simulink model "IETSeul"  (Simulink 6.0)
settings: Solver=ode45  StartTime=0.0  StopTime=SimTime  FixedStep=1E-2  RelTol=1e-5
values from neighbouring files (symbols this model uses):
  beta = 1    [ResCourV1.m]    (also in ResCrV1.m; ResEnerV1.m; Constantes.m = 0.95; ConstantesBck.m = 0.95)
  Cdl = 731.3E-9    (= 7.313e-07)    [ResCourV1.m]    (also in ResCrV1.m; ResEnerV1.m; Constantes.m = 6.03e-07; ConstantesBck.m = 6.03e-07)
  Cmem = 1E-6*Sm*(1-b)    (= 2.826e-08)    [Constantes.m]    (also in ConstantesBck.m = 3.14e-11; ImpedanceZtissus.m = 4e-08; Ztissus.m = 4e-08; CalculCharge.m = 1)
  I0Stim = AddI    (= 0)    [WaveComp.m]    (also in WaveCompIET.m; WaveCompIETAnim.m; WaveCompIETIf.m; WaveCompIETSeul.m = Hm(i)*1E-6)
  Rcan = 6.398E3*Sm*(1-b)    (= 180.80748)    [Constantes.m]    (also in ConstantesBck.m = 0.03454; ImpedanceZtissus.m = 44; Ztissus.m = 44)
  Rct = 605.2E3    (= 605200)    [ResCourV1.m]    (also in ResCrV1.m; ResEnerV1.m; Constantes.m = 185600; ConstantesBck.m = 185600)
  sigma = 68000    [ResCourV1.m]    (also in ResCrV1.m; ResEnerV1.m; Constantes.m = 66466; ConstantesBck.m = 66466)
  T0Stim = i    [WaveComp.m]    (also in WaveCompIET.m; WaveCompIETAnim.m = 5; WaveCompIETIf.m; WaveCompIETSeul.m = T0Hm(i)*1E-3)
  TypeStim = 5    [WaveComp.m]    (also in WaveCompIET.m; WaveCompIETAnim.m; WaveCompIETIf.m; WaveCompIETSeul.m)
libraries: simulink x1

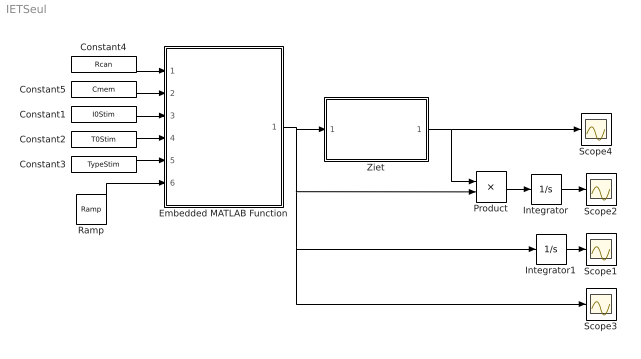
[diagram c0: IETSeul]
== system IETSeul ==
  Constant1 : Constant  Value=I0Stim
  Constant2 : Constant  Value=T0Stim
  Constant3 : Constant  Value=TypeStim
  Constant4 : Constant  Value=Rcan
  Constant5 : Constant  Value=Cmem
  Embedded MATLAB Function : Stateflow chart
  Integrator : Integrator
  Integrator1 : Integrator
  Product : Product
  Ramp : simulink/Sources/Ramp  slope=1  start=0  X0=0
  Scope{1..4} (4 alike) : Scope
  Ziet : Subsystem
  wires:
  Product/1 -> Integrator/1
  Constant1/1 -> Embedded MATLAB Function/3(I0Stim)
  Constant2/1 -> Embedded MATLAB Function/4(T0Stim)
  Constant3/1 -> Embedded MATLAB Function/5(TypeStim)
  Integrator1/1 -> Scope1/1
  Ramp/1 -> Embedded MATLAB Function/6(temps)
  Embedded MATLAB Function/1(Istim) -> Scope3/1, Integrator1/1, Product/2, Ziet/1(InZiet)
  Constant4/1 -> Embedded MATLAB Function/1(Rcan)
  Constant5/1 -> Embedded MATLAB Function/2(Cmem)
  Integrator/1 -> Scope2/1
  Ziet/1(OutZiet) -> Product/1, Scope4/1

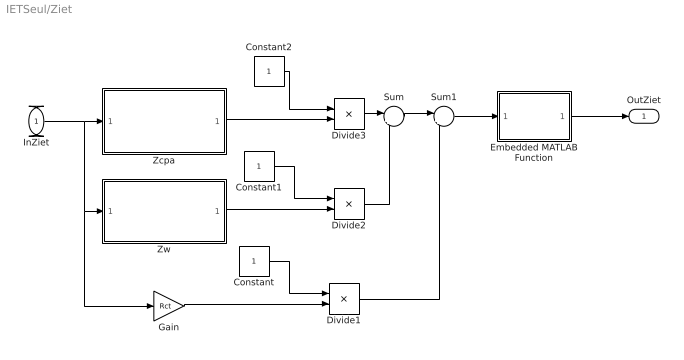
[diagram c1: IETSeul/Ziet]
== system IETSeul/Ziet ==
  InZiet : Inport  Port=1  LatchInput=off
  Constant : Constant
  Constant1 : Constant
  Constant2 : Constant
  Divide1 : Product  Inputs=*/  OutScaling=2^-10
  Divide2 : Product  Inputs=*/  OutScaling=2^-10
  Divide3 : Product  Inputs=*/  OutScaling=2^-10
  Embedded MATLAB Function : Stateflow chart
  Gain : Gain  Gain=Rct
  Sum : Sum  Inputs=|++
  Sum1 : Sum  Inputs=|++
  Zcpa : Subsystem
  Zw : Subsystem
  OutZiet : Outport
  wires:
  Constant/1 -> Divide1/1
  Constant1/1 -> Divide2/1
  Constant2/1 -> Divide3/1
  Zcpa/1(OutZcpa) -> Divide3/2
  Zw/1(OutZw) -> Divide2/2
  Divide3/1 -> Sum/1
  Divide2/1 -> Sum/2
  Sum/1 -> Sum1/1
  Divide1/1 -> Sum1/2
  Sum1/1 -> Embedded MATLAB Function/1(u)
  Gain/1 -> Divide1/2
  InZiet/1 -> Zcpa/1(InZcpa), Zw/1(InZw), Gain/1
  Embedded MATLAB Function/1(y) -> OutZiet/1

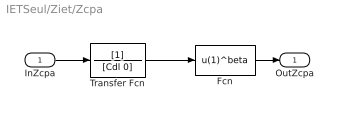
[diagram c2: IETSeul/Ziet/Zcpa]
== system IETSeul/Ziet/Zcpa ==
  InZcpa : Inport  Port=1  LatchInput=off
  Fcn : Fcn  Expr=u(1)^beta
  Transfer Fcn : TransferFcn  Denominator=[Cdl 0]
  OutZcpa : Outport
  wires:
  Transfer Fcn/1 -> Fcn/1
  InZcpa/1 -> Transfer Fcn/1
  Fcn/1 -> OutZcpa/1

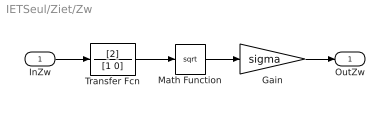
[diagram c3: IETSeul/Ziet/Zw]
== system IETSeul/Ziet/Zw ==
  InZw : Inport  Port=1  LatchInput=off
  Gain : Gain  Gain=sigma
  Math Function : Math  Operator=sqrt
  Transfer Fcn : TransferFcn  Numerator=[2]  Denominator=[1 0]
  OutZw : Outport
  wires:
  Transfer Fcn/1 -> Math Function/1
  Math Function/1 -> Gain/1
  Gain/1 -> OutZw/1
  InZw/1 -> Transfer Fcn/1

== matlab function Ziet/Embedded
MATLAB Function ==
function y = fcn(u)
% This block supports an embeddable subset of the MATLAB language.
% See the help menu for details. 

if u == Inf 
    y = 0;
else
    y = 1/u;
end

== matlab function Embedded
MATLAB Function ==
function Istim = courant(Rcan,Cmem,I0Stim,T0Stim,TypeStim,temps)
% This block supports an embeddable subset of the MATLAB language.
% See the help menu for details. 
taum = 1/30.4E-3*1E-6*1000;
if temps <= T0Stim
    if TypeStim == 0
        Iout = I0Stim;
    elseif TypeStim == 1
        Iout = I0Stim*exp(temps/taum);
    elseif TypeStim == 2
        Iout = I0Stim*sin(pi/T0Stim*temps);
    elseif TypeStim == 3
        Iout = I0Stim*sin(pi/(2*T0Stim)*temps);
    elseif TypeStim == 4
        Iout = I0Stim*sinh(temps/taum);
    else
        Iout = I0Stim*(sin(pi/T0Stim*temps)+1/3*sin(3*pi/T0Stim*temps));
    end
else
    Iout = 0;
end
Istim = Iout;
